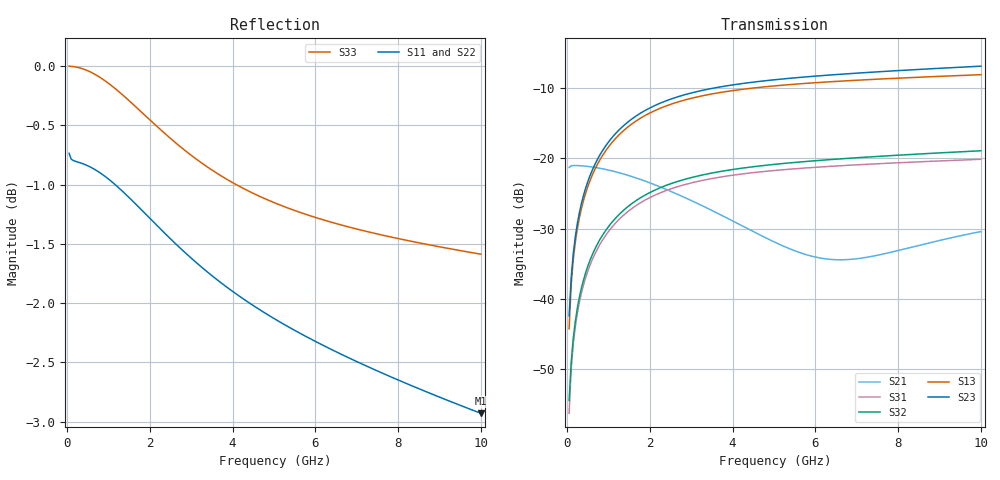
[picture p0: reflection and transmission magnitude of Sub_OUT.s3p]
! Created Wed Jul 11 12:20:10 2018
# ghz S ma R 50
! 3 Port Network Data from SP1.SP block
! freq  magS11  angS11  magS12  angS12  magS13  angS13
!  magS21  angS21
!  magS22  angS22  magS23  angS23
!  magS31  angS31  magS32  angS32
!  magS33  angS33
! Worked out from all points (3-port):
!   200 points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, 50 MHz to 10 GHz, reference 50 ohm
!   strongest paths, dB at 50 MHz, 2.55 GHz, 5.05 GHz, 7.55 GHz, 10 GHz:
!     S23: -42.4, -11.5, -8.8, -7.7, -6.9
!     S13: -44.3, -12.2, -9.7, -8.7, -8.1
!     S32: -54.5, -23.5, -20.8, -19.7, -18.9
!     S31: -56.3, -24.3, -21.7, -20.8, -20.1
!     S21: -21.3, -24.8, -32.0, -33.7, -30.4
!   lowest |S11| = -2.9 dB at 10 GHz (marker M1), VSWR 5.99, Z = 153 - j145 ohm
!   |S11| at or under -10 dB: nowhere
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0.05  0.9188 -1.7  0.08593 14.4  0.00612 105.0
      0.08593 14.4  0.9154 -1.8  0.007564 76.1
      0.00153 105.0  0.001891 76.1  0.9999 -0.2
0.1  0.9136 -1.3  0.08838 5.1  0.01259 96.3
     0.08838 5.1  0.91 -1.4  0.01413 80.9
     0.003148 96.3  0.003533 80.9  0.9998 -0.4
0.15  0.9124 -1.3  0.08878 1.0  0.01898 92.7
      0.08878 1.0  0.9087 -1.4  0.02088 82.4
      0.004745 92.7  0.00522 82.4  0.9996 -0.6
0.35  0.91 -2.0  0.08837 -8.0  0.04419 86.0
      0.08837 -8.0  0.9063 -2.2  0.04796 81.8
      0.01105 86.0  0.01199 81.8  0.9978 -1.3
0.65  0.9049 -3.4  0.08628 -17.7  0.0807 79.7
      0.08628 -17.7  0.9011 -3.8  0.08743 77.7
      0.02018 79.7  0.02186 77.7  0.9926 -2.4
1.1  0.8932 -5.3  0.08114 -30.8  0.1309 71.8
     0.08114 -30.8  0.8893 -6.0  0.1418 71.1
     0.03273 71.8  0.03546 71.1  0.9804 -3.8
2.5  0.8455 -9.7  0.05825 -66.1  0.2418 53.8
     0.05825 -66.1  0.8409 -11.1  0.2632 54.9
     0.06045 53.8  0.0658 54.9  0.9321 -6.3
5.05  0.7816 -13.7  0.02503 -128.8  0.3281 38.6
      0.02503 -128.8  0.7762 -16.5  0.3629 41.5
      0.08202 38.6  0.09071 41.5  0.8751 -7.3
6.75  0.754 -15.7  0.01898 172.9  0.3558 34.6
      0.01898 172.9  0.7483 -19.4  0.3988 38.2
      0.08895 34.6  0.09969 38.2  0.8558 -7.5
10  0.7137 -19.1  0.03007 108.9  0.3933 31.5
    0.03007 108.9  0.7077 -24.5  0.4522 36.0
    0.09833 31.5  0.113 36.0  0.833 -8.1
